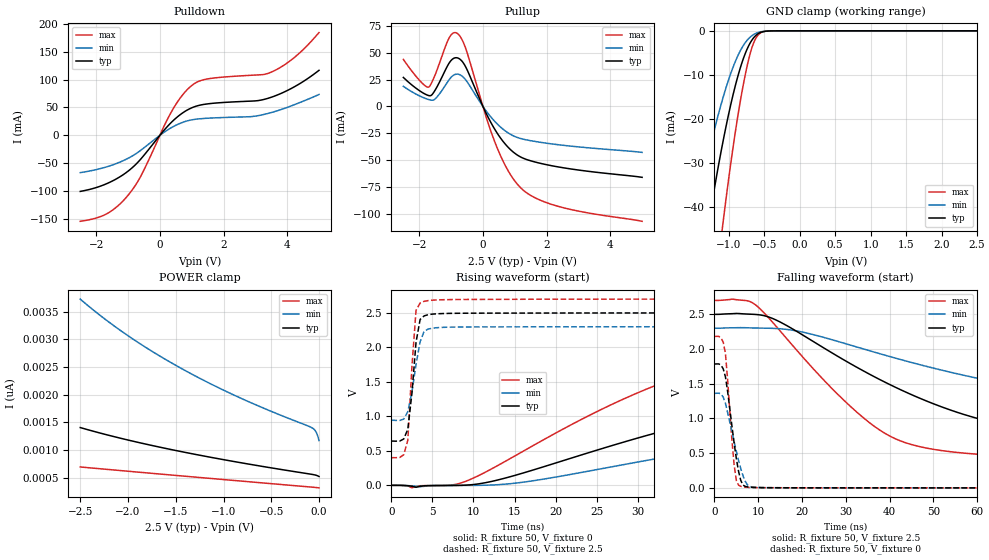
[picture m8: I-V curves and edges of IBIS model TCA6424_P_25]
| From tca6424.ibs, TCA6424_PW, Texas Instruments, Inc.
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[Model]   TCA6424_P_25
Model_type  I/O
Vinl=0.69
Vinh=1.89
Enable   Active-Low
Vref =   0
Rref =   500
Cref =   50p
Vmeas =   1.25
| variable   typ   min   max
C_comp   3.69pF   2.93pF   4.10pF
| C_pullup   6.79pF   2.74pF   10.86pF
| C_pulldown   4.46pF   3.36pF   6.24pF
| C_tri-state   3.69pF   2.93pF   4.10pF
[Temperature Range]   40   100   -40
| Ambient temperature   25   85   -40
[Voltage range]   2.5   2.3   2.7
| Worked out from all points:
|   slope of the pulldown table from 0 to 0.375 V, typ, clamps not added: 15.6 ohm
|   slope of the pullup table from 0 to 0.375 V, typ, clamps not added: 17.4 ohm
|   GND clamp passes 1 mA (typ) near -0.61 V on its own axis
|   rising waveform, R_fixture 50, V_fixture 0: 20-80 % time 39.1ns typ, 55.9ns min, 24.3ns max; typ from 0 V to 1.78 V
|   falling waveform, R_fixture 50, V_fixture 2.5: 20-80 % time 37.3ns typ, 65.3ns min, 21.8ns max; typ from 2.5 V to 0.642 V
|   rising waveform, R_fixture 50, V_fixture 2.5: 20-80 % time 889ps typ, 1.16ns min, 722ps max; typ from 0.642 V to 2.5 V
|   falling waveform, R_fixture 50, V_fixture 0: 20-80 % time 2.26ns typ, 3.04ns min, 1.59ns max; typ from 1.78 V to 0 V
[GND Clamp]
| TCA6424_P_25
|   Voltage   I(typ)   I(min)   I(max)
-2.5V     -199.5mA   -143mA     -290.2mA
-1.495V   -66.41mA   -44.03mA   -105.9mA
-1.3V     -45.47mA   -29.17mA   -74.94mA
-1.275V   -42.97mA   -27.43mA   -71.16mA
-1.085V   -25.59mA   -15.5mA    -44.34mA
-960mV    -16.02mA   -9.208mA   -28.93mA
-830mV    -8.107mA   -4.347mA   -15.43mA
-720mV    -3.455mA   -1.786mA   -6.597mA
-635mV    -1.338mA   -725.2uA   -2.246mA
-555mV    -393.8uA   -252.8uA   -513.9uA
-435mV    -36.87uA   -30.65uA   -32.48uA
2.5V      522.1pA    1.492nA    -263.6pA
[POWER Clamp]
| TCA6424_P_25
|   Voltage   I(typ)   I(min)   I(max)
-2.5V     1.406nA    3.726nA    694pA
-2.3V     1.31nA     3.443nA    663pA
-2.095V   1.22nA     3.18nA     631.5pA
-1.87V    1.129nA    2.916nA    597.3pA
-1.635V   1.04nA     2.665nA    561.8pA
-1.295V   921.5pA    2.337nA    510.7pA
-930mV    804.6pA    2.025nA    456.2pA
-560mV    694.8pA    1.742nA    401.3pA
-80mV     562pA      1.408nA    330.3pA
-35mV     546.4pA    1.339nA    323pA
-15mV     534.7pA    1.261nA    319.4pA
-31.15fV  522.1pA    1.17nA     316.6pA
[Pulldown]
| TCA6424_P_25
|   Voltage   I(typ)   I(min)   I(max)
-2.5V     -100.3mA   -66.72mA   -153.8mA
-1.665V   -86.32mA   -56.23mA   -140.3mA
-995mV    -63.91mA   -40.95mA   -107mA
-580mV    -41.14mA   -25.84mA   -71.06mA
400mV     25.38mA    15.01mA    45.82mA
705mV     39.76mA    23.05mA    71.75mA
1.005V    49.41mA    27.82mA    89.36mA
1.53V     56.6mA     30.79mA    101.3mA
2.88V     61.37mA    33.64mA    107.6mA
3.48V     67.85mA    40.52mA    112.8mA
4.23V     87.1mA     55.01mA    139.6mA
5V        116.4mA    73.18mA    184mA
[Pullup]
| TCA6424_P_25
|   Voltage   I(typ)   I(min)   I(max)
-2.5V     27.05mA    18.71mA    43.88mA
-1.705V   10.14mA    6.404mA    18.04mA
-1.495V   15.53mA    7.156mA    29.94mA
-1.065V   40.3mA     24.79mA    63.75mA
-805mV    45.35mA    30.16mA    68.19mA
-535mV    36.51mA    24.55mA    53.62mA
105mV     -6.664mA   -4.379mA   -10.22mA
445mV     -24.83mA   -16.25mA   -38.52mA
805mV     -38.57mA   -24.98mA   -60.74mA
1.17V     -46.99mA   -29.85mA   -75.51mA
2.36V     -56.47mA   -35.74mA   -93.28mA
5V        -66.2mA    -42.93mA   -107.3mA
[Ramp]
| TCA6424_P_25
| variable   typ   min   max
dV/dt_r   1.09/3.93E-08   0.83/5.61E-08   1.33/2.46E-08
dV/dt_f   1.12/3.74E-08   0.82/6.54E-08   1.39/2.19E-08
R_load = 50
[Rising Waveform]
| TCA6424_P_25
R_fixture =   50
C_fixture =   0
L_fixture =   0
V_fixture =   0
V_fixture_min = 0
V_fixture_max = 0
|   Time   V(typ)   V(min)   V(max)
0s        1.68nV     12.67nV    504.7pV
9ns       2.519mV    -1.473mV   55.94mV
16ns      177mV      44.79mV    491mV
27.5ns    598.7mV    282.8mV    1.209V
40ns      995.2mV    542.7mV    1.762V
50.5ns    1.252V     725.2mV    1.987V
65.5ns    1.504V     926.8mV    2.099V
103ns     1.718V     1.206V     2.167V
156ns     1.773V     1.325V     2.181V
520ns     1.784V     1.361V     2.182V
[Falling Waveform]
| TCA6424_P_25
R_fixture =   50
C_fixture =   0
L_fixture =   0
V_fixture =   2.5
V_fixture_min = 2.3
V_fixture_max = 2.7
|   Time   V(typ)   V(min)   V(max)
0s        2.5V       2.3V       2.7V
9.5ns     2.498V     2.303V     2.631V
15ns      2.39V      2.292V     2.261V
28ns      1.901V     2.114V     1.358V
39ns      1.521V     1.911V     783.6mV
47ns      1.289V     1.774V     592.1mV
60.5ns    993.3mV    1.573V     482.8mV
92ns      733mV      1.256V     419.7mV
162ns     651mV      1.006V     402.6mV
520ns     642mV      944.6mV    401.5mV
[Rising Waveform]
| TCA6424_P_25
R_fixture =   50
C_fixture =   0
L_fixture =   0
V_fixture =   2.5
V_fixture_min = 2.3
V_fixture_max = 2.7
|   Time   V(typ)   V(min)   V(max)
0s        642mV      944.5mV    401.5mV
1ns       641.2mV    940.2mV    403.8mV
1.5ns     672.1mV    960.9mV    442.7mV
2ns       812.6mV    1.068V     654.7mV
2.5ns     1.335V     1.353V     1.719V
3ns       2.074V     1.753V     2.537V
3.5ns     2.406V     2.083V     2.644V
4ns       2.458V     2.237V     2.669V
6ns       2.49V      2.289V     2.69V
520ns     2.5V       2.3V       2.7V
[Falling Waveform]
| TCA6424_P_25
R_fixture =   50
C_fixture =   0
L_fixture =   0
V_fixture =   0
V_fixture_min = 0
V_fixture_max = 0
|   Time   V(typ)   V(min)   V(max)
0s        1.784V     1.361V     2.182V
1.5ns     1.767V     1.351V     2.161V
2ns       1.715V     1.308V     2.099V
2.5ns     1.599V     1.219V     1.937V
4ns       884.2mV    803.3mV    671.8mV
4.5ns     638.8mV    661.7mV    324.7mV
5ns       419.2mV    524.6mV    105.8mV
6ns       107.5mV    277.5mV    22.03mV
7.5ns     14.57mV    45.42mV    7.227mV
520ns     81.62nV    304.4nV    43.18nV
